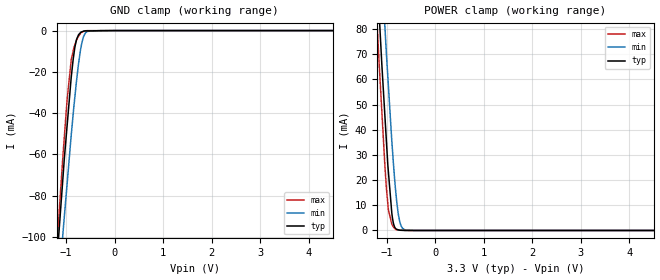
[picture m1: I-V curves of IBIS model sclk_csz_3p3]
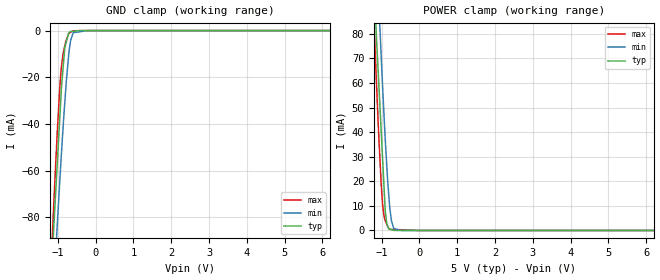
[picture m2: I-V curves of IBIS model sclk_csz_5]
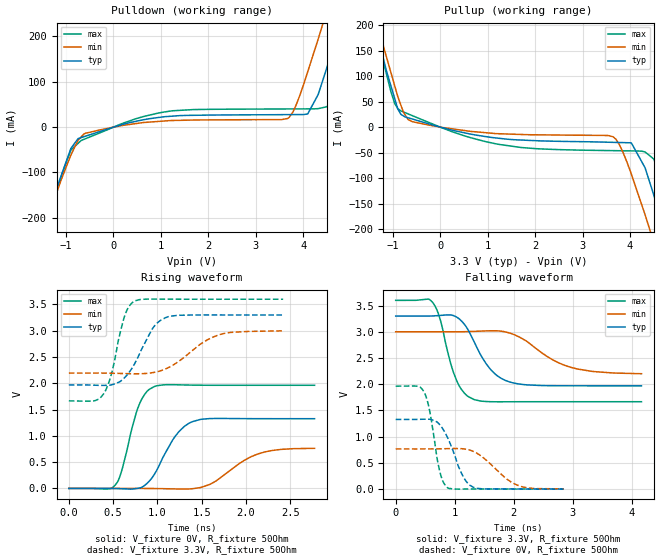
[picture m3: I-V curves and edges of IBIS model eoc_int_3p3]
|Texas Instruments Incorporated
|Serial Out, Low Power with Built-In Conversion Clock & 8x FIFO, 4 Channels
| Marketing part#   Digital Voltage Range   Package-type   #pins
| TLC3574IDW   2.7V - 5.5V   SOIC   20
| TLC3574IDWG4   2.7V - 5.5V   SOIC   20
| TLC3574IDWR   2.7V - 5.5V   SOIC   20
| TLC3574IDWRG4   2.7V - 5.5V   SOIC   20
| TLC3574IPW   2.7V - 5.5V   TSSOP   20
| TLC3574IPWG4   2.7V - 5.5V   TSSOP   20
[IBIS Ver]   4.0
[File name]   tlc3574.ibs
[File Rev]   1.0
[Date]   1/10/2012
[Source]
| Texas Instruments Incorporated.
| Analog-eLab Design Center, HPA
| 12500 TI Blvd
| Dallas, TX -75243
| e-mail: elab_scm_ibis@list.ti.com
[Notes]   Revision History:
| Rev 1.0: 1/10/2012
| - Initial version of the model
| - Model generated from simulations in TISPICE
| - Model matched to SPICE simulation
| - C_comp although listed in numerical order of value are
|   obtained from varying PVT conditions. For PVT conditions for
|   each specific value refer the buffer description under
|   respective [Model]. IBIS model user is responsible for using
|   appropriate C_comp to simulate for Signal Integrity.
| - Model names with a trailing _3p3 contains the model for
|   3.3V [3.0V and 3.6V]. Model names with a trailing _5 contains
|   the model for 5.0V [4.5V and 5.5V].
[Disclaimer]
| This model is designed as an aid for customers of Texas Instruments.
| TI and its licensors and suppliers make no warranties, either expressed
| or implied, with respect to this  model, including the warranties of
| merchantability or fitness for a particular purpose. The model is
| provided solely on an "as is" basis. The entire risk as to its quality
| and performance is with the customer.
[Copyright]
 (C) Copyright 2012 Texas Instruments Incorporated.All rights reserved.
|   TLC3574DW
[Component]   TLC3574DW
[Manufacturer]   TI
[Package]   |20 SOIC   -  DW package
|   typ   min   max
R_pkg   0.11471   0.09873   0.13721
L_pkg   3.77779nH   2.82917nH   4.54063nH
C_pkg   0.71510pF   0.50156pF   0.93260pF
[Pin]  signal_name   model_name   R_pin   L_pin   C_pin
1   SCLK   SCLK_CSZ   0.11628   4.54063nH  0.93249pF
2   FS   INPUT   0.12052   4.08328nH  0.76195pF
3   SDI   INPUT   0.13721   3.54797nH  0.59198pF
4   EOC/_INT   EOC_INT   0.09990   3.05073nH  0.55007pF
5   SDO   SDO   0.10034   2.82927nH  0.50156pF
6   DGND   GND   0.05254   2.43837nH  0.54492pF
7   DVDD   POWER   0.05782   2.85070nH  0.60072pF
8   _CS   SCLK_CSZ   0.13377   3.48857nH  0.58803pF
9   A0   TERM   0.11957   4.07378nH  0.76123pF
10   A1   TERM   0.11419   4.50963nH  0.93137pF
11   A2   TERM   0.11446   4.51493nH  0.93163pF
12   A3   TERM   0.12001   4.08228nH  0.76153pF
13   AVDD   POWER   0.13381   3.48937nH  0.58791pF
14   AGND   GND   0.05641   2.75326nH  0.59922pF
15   REFP   TERM   0.10030   2.82917nH  0.50302pF
16   REFM   GND   0.09748   2.77397nH  0.49914pF
17   COMP   TERM   0.09873   3.02783nH  0.54884pF
18   AGND   GND   0.13622   3.52847nH  0.59030pF
19   AVDD   POWER   0.12094   4.09148nH  0.76228pF
20   _CSTART   INPUT   0.11589   4.53323nH  0.93260pF
|   TLC3574PW
[Component]   TLC3574PW
[Manufacturer]   TI
[Package]   |20 TSSOP  -  PW package
|   typ   min   max
R_pkg   0.07911   0.06722   0.08929
L_pkg   1.27417nH   1.03620nH   1.49755nH
C_pkg   0.13638pF   0.12233pF   0.14813pF
[Pin]  signal_name   model_name   R_pin   L_pin   C_pin
1   SCLK   SCLK_CSZ   0.08929   1.49755nH  0.14694pF
2   FS   INPUT   0.08576   1.38000nH  0.14694pF
3   SDI   INPUT   0.06879   1.06280nH  0.12484pF
4   EOC/_INT   EOC_INT   0.06929   1.07125nH  0.12498pF
5   SDO   SDO   0.07017   1.08905nH  0.12268pF
6   DGND   GND   0.04333   0.91001nH  0.15621pF
7   DVDD   POWER   0.04700   1.03908nH  0.16445pF
8   _CS   SCLK_CSZ   0.06722   1.03620nH  0.12233pF
9   A0   TERM   0.08609   1.39123nH  0.14735pF
10   A1   TERM   0.08693   1.46341nH  0.14564pF
11   A2   TERM   0.08759   1.47512nH  0.14613pF
12   A3   TERM   0.08663   1.40171nH  0.14813pF
13   AVDD   POWER   0.06739   1.03760nH  0.12268pF
14   AGND   GND   0.04571   0.95682nH  0.16273pF
15   REFP   TERM   0.07461   1.17220nH  0.12782pF
16   REFM   GND   0.06751   1.04235nH  0.11969pF
17   COMP   TERM   0.06754   1.04078nH  0.12260pF
18   AGND   GND   0.06770   1.04343nH  0.12290pF
19   AVDD   POWER   0.08625   1.39223nH  0.14765pF
20   _CSTART   INPUT   0.08858   1.48294nH  0.14659pF
1000   THERMAL_PAD   NC   0.00006   0.00136nH  1.25128pF
|   Model Selectors
[Model Selector] SCLK_CSZ
sclk_csz_3p3  3.3V digital input
sclk_csz_5   5.0V digital input
[Model Selector] INPUT
input_3p3  3.3V digital input
input_5   5.0V digital input
[Model Selector] EOC_INT
eoc_int_3p3  3.3V digital output
eoc_int_5   5.0V digital output
[Model Selector] SDO
sdo_3p3  3.3V digital 3-state
sdo_5   5.0V digital 3-state
[Model Selector] TERM
term_3-3V  3.3V nominal termination
term_5-0V  5.0V nominal termination
[Model] term_3-3V
Model_type Terminator
C_comp   1.0e-20F  1.0e-20F  1.0e-20F
|   typ   min   max
[Voltage Range]   3.3V   3.0V   3.6V
[POWER Clamp Reference]   3.3V   3.0V   3.6V
[GND Clamp Reference]   0V   0V   0V
|Ambient Temperature   25   85   -40
|Junction Temperature
[Temperature Range]   27   125   -40
[Model] term_5-0V
Model_type Terminator
C_comp   1.0e-20F  1.0e-20F  1.0e-20F
|   typ   min   max
[Voltage Range]   5.0V   4.5V   5.5V
[POWER Clamp Reference]   5.0V   4.5V   5.5V
[GND Clamp Reference]   0V   0V   0V
|Ambient Temperature   25   85   -40
|Junction Temperature
[Temperature Range]   27   125   -40
| Models and submodels in the file (10): sclk_csz_3p3 (Input), sclk_csz_5 (Input), input_3p3 (Input), input_5 (Input), eoc_int_3p3 (Output), eoc_int_5 (Output), sdo_3p3 (3-state), sdo_5 (3-state), term_3-3V (Terminator), term_5-0V (Terminator)
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|   sclk_csz_3p3 Model
[Model]   sclk_csz_3p3
Model_type   Input
Vinl = 0.6
Vinh = 2.1
|   typ   min   max
C_comp   1.035e-12   1.031e-12   1.043e-12
[Voltage Range]   3.3   3   3.6
|Ambient Temperature   25   85   -40
|Junction Temperature
[Temperature Range]   27   125   -40
[Power Clamp Reference]   3.3   3   3.6
[GND Clamp Reference]   0   0   0
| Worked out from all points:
|   GND clamp passes 1 mA (typ) near -0.71 V on its own axis
|   POWER clamp passes 1 mA (typ) near -0.83 V on its own axis
[GND Clamp]
|   Voltage   I(typ)   I(min)   I(max)
-3.3V     -917.7mA   -878.5mA   -974mA
-1.228V   -122.7mA   -146.6mA   -117.7mA
-1.116V   -86.8mA    -112.5mA   -77.29mA
-1.062V   -69.45mA   -96.55mA   -58.73mA
-982.8mV  -46.36mA   -74.5mA    -33.74mA
-896.4mV  -22.48mA   -50.46mA   -14.1mA
-858mV    -14.11mA   -40.68mA   -10.02mA
-792mV    -4.734mA   -25.23mA   -4.892mA
-696.3mV  -771.6uA   -8.202mA   -1.071mA
-591mV    -162uA     -855.5uA   -65.11uA
-285mV    -77.64uA   -291.2nA   -96.65nA
6.6V      0A         0A         0A
[POWER Clamp]
|   Voltage   I(typ)   I(min)   I(max)
-3.3V     944.2mA    958.8mA    947.2mA
-1.294V   135.3mA    171.8mA    117.7mA
-1.158V   85.84mA    121.6mA    66mA
-1.105V   66.7mA     103.5mA    47.99mA
-1.037V   44.38mA    79.7mA     24.57mA
-968.4mV  23.3mA     57.46mA    8.167mA
-897.6mV  6.816mA    35.48mA    2.469mA
-810mV    592.7uA    13.98mA    336.9uA
-762mV    230.6uA    6.263mA    214.6uA
-711mV    72.54uA    2.038mA    122.9uA
-591mV    14.36uA    100.7uA    17.6uA
6.6V      0A         0A         0A
|   sclk_csz_5 Model
[Model]   sclk_csz_5
Model_type   Input
Vinl = 0.8
Vinh = 3.8
|   typ   min   max
C_comp   9.450e-13   9.377e-13   9.523e-13
[Voltage Range]   5   4.5   5.5
|Ambient Temperature   25   85   -40
|Junction Temperature
[Temperature Range]   27   125   -40
[Power Clamp Reference]   5   4.5   5.5
[GND Clamp Reference]   0   0   0
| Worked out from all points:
|   GND clamp passes 1 mA (typ) near -0.71 V on its own axis
|   POWER clamp passes 1 mA (typ) near -0.82 V on its own axis
[GND Clamp]
|   Voltage   I(typ)   I(min)   I(max)
-5V       -1.611A    -1.528A    -1.703A
-1.14V    -93.77mA   -120.4mA   -86.32mA
-1.111V   -85.23mA   -111.5mA   -75.54mA
-1.018V   -57.68mA   -83.96mA   -44.24mA
-951.5mV  -38.23mA   -65.2mA    -25.23mA
-907.5mV  -25.27mA   -53.4mA    -15.85mA
-815mV    -7.17mA    -30.66mA   -6.526mA
-711mV    -1.061mA   -10.14mA   -1.388mA
-670mV    -439.4uA   -5.093mA   -734.4uA
-594mV    -297.5uA   -921.6uA   -60.21uA
-202.5mV  -317.9nA   -28.16nA   -20.53uA
10V       0A         0A         0A
[POWER Clamp]
|   Voltage   I(typ)   I(min)   I(max)
-5V       1.663A     1.661A     1.686A
-1.373V   166.4mA    200.6mA    151mA
-1.144V   81.22mA    117mA      63.01mA
-1.067V   57.57mA    90.09mA    36.02mA
-1.012V   40.88mA    71.5mA     19.36mA
-973.5mV  29.19mA    58.73mA    10.65mA
-900mV    7.533mA    36.19mA    3.846mA
-797.5mV  591.4uA    11.94mA    486.5uA
-738mV    324uA      3.807mA    450.2uA
-679.5mV  61.04uA    938.6uA    414.5uA
-477mV    6.782uA    4.775uA    291uA
10V       0A         0A         0A
|   eoc_int_3p3 Model
[Model]   eoc_int_3p3
Model_type   Output
Polarity   Non-Inverting
Vmeas = 1.65
Vref = 1.65
Cref = 10pF
Rref = 50
|   typ   min   max
C_comp   1.501e-12   1.479e-12   1.546e-12
| Where nom  PVT is Nominal Process, 3.3V, 27C
|   Fast PVT is Strong Process,  3.6V, -40C
|   Slow PVT is Weak Process,   3V, 125C
[Voltage Range]   3.3   3   3.6
|Ambient Temperature   25   85   -40
|Junction Temperature
[Temperature Range]   27   125   -40
[Pullup Reference]   3.3   3   3.6
[Pulldown Reference]   0   0   0
[Power Clamp Reference]   3.3   3   3.6
[GND Clamp Reference]   0   0   0
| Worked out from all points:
|   slope of the pulldown table from 0 to 0.495 V, typ, clamps not added: 37.2 ohm
|   slope of the pullup table from 0 to 0.495 V, typ, clamps not added: 45.5 ohm
|   falling waveform, V_fixture 3.3V, R_fixture 50Ohm: 20-80 % time 419ps typ, 676ps min, 279ps max; typ from 3.3 V to 1.97 V
|   rising waveform, V_fixture 0V, R_fixture 50Ohm: 20-80 % time 269ps typ, 398ps min, 182ps max; typ from 0 V to 1.33 V
|   rising waveform, V_fixture 3.3V, R_fixture 50Ohm: 20-80 % time 250ps typ, 392ps min, 159ps max; typ from 1.97 V to 3.3 V
|   falling waveform, V_fixture 0V, R_fixture 50Ohm: 20-80 % time 288ps typ, 460ps min, 175ps max; typ from 1.33 V to 0 V
[Pulldown]
|   Voltage   I(typ)   I(min)   I(max)
-3.3V     -905.2mA   -842.3mA   -981.7mA
-1.458V   -223.6mA   -222mA     -241.7mA
-896.4mV  -46.97mA   -61.39mA   -50.41mA
-591mV    -19.98mA   -13.53mA   -25.59mA
1.073V    22.91mA    13.55mA    33.44mA
3.675V    27.6mA     19.12mA    40.1mA
3.855V    27.71mA    49.66mA    40.17mA
4.095V    28.94mA    121.9mA    40.26mA
4.468V    120.7mA    246mA      44.25mA
4.662V    190mA      313.5mA    80.72mA
5.054V    332mA      454mA      220.3mA
6.6V      919.2mA    1.025A     824.2mA
[Pullup]
|   Voltage   I(typ)   I(min)   I(max)
-3.3V     944.1mA    936.5mA    967.9mA
-1.368V   195.6mA    217.6mA    190mA
-961.2mV  55.83mA    80.81mA    46.25mA
-591mV    15.95mA    10.76mA    22.54mA
1.246V    -21.94mA   -12.94mA   -33.94mA
3.642V    -29.81mA   -18.9mA    -46.05mA
4.029V    -31.19mA   -92.54mA   -46.58mA
4.468V    -123.4mA   -216.2mA   -60.05mA
4.709V    -201.1mA   -292mA     -118.5mA
4.871V    -253.9mA   -343.6mA   -174.2mA
5.123V    -342.5mA   -423.7mA   -266.7mA
6.6V      -890.8mA   -927.5mA   -852.4mA
[Ramp]
R_load = 50
|   typ   min   max
dV/dt_r   0.796087/2.6868e-10   0.458802/3.98101e-10   1.17761/1.82295e-10
dV/dt_f   0.798477/4.18392e-10   0.482832/6.80875e-10   1.16051/2.79318e-10
[Falling Waveform]
V_fixture = 3.3V
V_fixture_min = 3V
V_fixture_max = 3.6V
R_fixture = 50Ohm
|   Time   V(typ)   V(min)   V(max)
0s        3.3V       3V         3.6V
625ps     3.302V     3V         3.562V
750ps     3.311V     3V         3.252V
930ps     3.322V     3V         2.403V
1.03ns    3.282V     3V         2.077V
1.33ns    2.806V     3.008V     1.707V
1.635ns   2.249V     3.019V     1.666V
1.985ns   2.026V     2.955V     1.665V
2.965ns   1.97V      2.323V     1.666V
4.165ns   1.969V     2.2V       1.666V
[Rising Waveform]
V_fixture = 0V
V_fixture_min = 0V
V_fixture_max = 0V
R_fixture = 50Ohm
|   Time   V(typ)   V(min)   V(max)
0s        187.1pV    574.5pV    162.6pV
525ps     -2.774mV   332.5uV    67.15mV
600ps     -6.561mV   397uV      353mV
795ps     7.359mV    -118.7uV   1.596V
965ps     265.2mV    -2.625mV   1.937V
1.2ns     989.6mV    -9.805mV   1.973V
1.4ns     1.272V     -4.843mV   1.965V
1.6ns     1.33V      82.71mV    1.963V
2.135ns   1.327V     655.8mV    1.962V
2.775ns   1.327V     763.2mV    1.963V
[Rising Waveform]
V_fixture = 3.3V
V_fixture_min = 3V
V_fixture_max = 3.6V
R_fixture = 50Ohm
|   Time   V(typ)   V(min)   V(max)
0s        1.969V     2.195V     1.665V
275ps     1.966V     2.195V     1.662V
400ps     1.961V     2.194V     1.819V
485ps     1.973V     2.191V     2.2V
625ps     2.099V     2.185V     3.255V
740ps     2.364V     2.181V     3.565V
955ps     3.065V     2.206V     3.602V
1.115ns   3.264V     2.291V     3.601V
1.7ns     3.3V       2.925V     3.6V
2.42ns    3.3V       2.998V     3.6V
[Falling Waveform]
V_fixture = 0V
V_fixture_min = 0V
V_fixture_max = 0V
R_fixture = 50Ohm
|   Time   V(typ)   V(min)   V(max)
0s        1.327V     764.8mV    1.963V
365ps     1.329V     764.5mV    1.961V
485ps     1.332V     764.7mV    1.846V
575ps     1.331V     765.2mV    1.497V
750ps     1.223V     767.3mV    324.9mV
885ps     967.1mV    770.4mV    20.52mV
1.135ns   257.6mV    767.9mV    -572.6uV
1.32ns    31.8mV     715.6mV    170.5uV
2.09ns    598.1uV    61.12mV    165.4uV
2.85ns    110.5uV    2.747mV    150.8uV
